| IBIS File LibisMaker.ibs
| Cadence Design Systems, Inc. 2024
|[Doc Num]	 FPGA-MD-02035 Ver 1.5
[IBIS ver]   4.2
[File name]   lfmxo5.ibs
[File Rev]   2.5.1
[Date]   Mon Jun 15 19:07:13 PDT 2026
[Source]   Lattice Semiconductor 28fdsoi Process
[Notes]   Device: LFMXO5-25
   BBG256   Final
   BBG400   Final
   Device: LFMXO5-100T
   BBG400   Final
   Device: LFMXO5-55T
   BBG400   Final
   Device: LFMXO5-15D
   BBG256   Final
   BBG400   Final
   Device: LFMXO5-55TD
   BBG400   Final
   Device: LFMXO5-55TDQ
   BBG400   Final
   CBG256   Final
   Device: LFMXO5-65TDQ
   BBG400   Final
   Device: LFMXO5-65T
   BBG256   Final
   BBG400   Final
   BBG484   Final
   Device: LFMXO5-65
   BBG256   Final
   BBG400   Final
   BBG484   Final
   Device: LFMXO5-35T
   BBG256   Final
   BBG400   Final
   BBG484   Final
   Device: LFMXO5-35
   BBG256   Final
   BBG400   Final
   BBG484   Final
   Device: LFMXO5-20D
   BBG256   Final
   BBG400   Final
   BBG484   Final
   Device: LFMXO5-20TD
   BBG256   Final
   BBG400   Final
   BBG484   Final
   Device: LFMXO5-20DQ
   BBG256   Final
   BBG400   Final
   BBG484   Final
   Device: LFMXO5-20TDQ
   BBG256   Final
   BBG400   Final
   BBG484   Final
   Device: LFMXO5-30D
   BBG256   Final
   BBG400   Final
   BBG484   Final
   Device: LFMXO5-30TD
   BBG256   Final
   BBG400   Final
   BBG484   Final
   Device: LFMXO5-30DQ
   BBG256   Final
   BBG400   Final
   BBG484   Final
   Device: LFMXO5-30TDQ
   BBG256   Final
   BBG400   Final
   BBG484   Final
   Lattice Semiconductor has worked hard to ensure the
   models below are accurate and complete.  However, the
   data below was generated using simulation of the
   input/output model files for the silicon.  Therefore,
   the data below is for reference and initial design
   purposes only.
   Lattice Semiconductor grants permission to use this
   data for use in printed circuit design using this
   Lattice programmable logic device.  Other use of this
   code, including the selling or duplication of any
   portion is strictly prohibited.
|   NAMING CONVENTION
   The IBIS [Model] header is limited by the specification to a
   total of characters.  With such a set of characters available
   for naming models it becomes important to attempt to
   meaningfully encode the IO standards so they fit within the
   twenty character limit.  It would seem that twenty characters
   would provide room enough for describing IO's.  However, the
   PLD IO structure continues to grow more and more complex.  The
   complexity is making the twenty characters insuffiently
   descriptive.  In order to overcome this issue the naming
   convention described below is implemented to resolve the issue.
The twenty character space is managed as follows:
   bbbvvvsdddprttmaoixx
   b = standard
   v = voltage (x.xx V)
   s = slew code
   d = drive (xx.x ma)
   p = pullmode code
   r = impedance
   t = termination code
   m = mipi hard dphy mode
   o = diff resistor code
   i = diff  current code
   x = reserved
   standard
   LVCMOS   lvc
   LVCMOSH   lvh
   LVCMOSR   lvr
   LVCMOSD   lvd
   LVTTL   lvt
   lvttld   ltd
   sstl_I   ss1
   sstl_II   ss2
   sstld_I   s1d
   sstld_II   s2d
   hsul   hs1
   hsuld   h1d
   hstl_I   hs1
   hstld_I   h1d
   lvds   lvs
   lvdse   lve
   SUBLVDS   slv
   sublvdse   sle
   sublvdseh   slh
   slvs   svs
   mipi   mip
   vref1   vr1
   lvstl_I   ll1
   lvstl_II   ll2
   lvstld_I   l1d
   lvstld_II   l2d
   slew
   na   a
   fast   f
   slow   s
   med   m
   drive
   2   020
   4   040
   6   060
   8   080
   10   100
   12   120
   16   160
   50rs   r50
   na   xxx
   pullmode/clamp on
   none   a/e
   failsafe   a/e
   up   b/f
   down   c/g
   keeper   d/h
   i3c   i
   impedance
   off   a
   termination
   off   aa
   40   bb
   50   cc
   60   dd
   75   ee
   150   ff
   48   gg
   80   hh
   120   ii
   mipi hard dphy mode
   off   a
   lp   l
   hs   h
   differential resistor
   off   a
   100   b
   differential current
   NA   a
   2.0   b
   3.5   c
   Reserved   IO type
   in   input only (mipi: rx)
   ou   output (mipi: tx)
   io   I/O
   od   Open drain
   ic   Inverting differential input
   (signal name only)
   it   Non-Inverting differential
   input (signal name only)
   on   Inverting differential output
   (signal name only)
   op   Non-Inverting differential output
   (signal name only)
   bn   Inverting differential I/O
   (signal name only)
   bp   Non-Inverting differential I/O
   (signal name only)
   All the IO models are generated with pull mode set to none.
   Lattice Semiconductor Corporation
   5555 NE Moore Court
   Hillsboro, OR 97214
   U.S.A
   TEL: 1-800-Lattice (USA and Canada)
   408-826-6000 (other locations)
   web: http://www.latticesemi.com/
   email: techsupport@latticesemi.com
[Disclaimer] This IBIS source code is intended as a design reference
   which illustrates how the Lattice Semiconductor device operates.
   It is the user's responsibility to verify their design for
   consistency and functionality through the use of formal
   verification methods.  Lattice Semiconductor provides no warranty
   regarding the use or functionality of this data.
[Copyright]   Copyright 2025 by Lattice Semiconductor Corporation
|   Component LFMXO5
[Component] LFMXO5
[Manufacturer] Lattice Semiconductor Corp.
[Package]
|BBG400_15D
| variable   typ   min   max
R_pkg   0.36549   0.21269   0.57866
L_pkg   3.644e-9   2.134e-9   6.024e-9
C_pkg   1.195e-12   7.084e-13   1.745e-12
|BBG400_15D-AQA
| variable   typ   min   max
|R_pkg   0.36549   0.21269   0.57866
|L_pkg   3.644e-9   2.134e-9   6.024e-9
|C_pkg   1.195e-12   7.084e-13   1.745e-12
|BBG400_15D-HBN
| variable   typ   min   max
|R_pkg   0.36549   0.21269   0.57866
|L_pkg   3.644e-9   2.134e-9   6.024e-9
|C_pkg   1.195e-12   7.084e-13   1.745e-12
|BBG256_15D
| variable   typ   min   max
|R_pkg   0.31029   0.20925   0.48462
|L_pkg   3.215e-9   2.242e-9   4.974e-9
|C_pkg   1.086e-12   7.406e-13   1.53e-12
|BBG400_25
| variable   typ   min   max
|R_pkg   0.36549   0.21269   0.57866
|L_pkg   3.644e-9   2.134e-9   6.024e-9
|C_pkg   1.195e-12   7.084e-13   1.745e-12
|BBG256_25
| variable   typ   min   max
|R_pkg   0.31029   0.20925   0.48462
|L_pkg   3.215e-9   2.242e-9   4.974e-9
|C_pkg   1.086e-12   7.406e-13   1.53e-12
|BBG256_35
| variable   typ   min   max
|R_pkg   0.36575   0.16548   0.7091
|L_pkg   3.369e-9   1.878e-9   5.893e-9
|C_pkg   1.068e-12   6.45e-13   1.798e-12
|BBG256_35T
| variable   typ   min   max
|R_pkg   0.36575   0.16548   0.7091
|L_pkg   3.369e-9   1.878e-9   5.893e-9
|C_pkg   1.068e-12   6.45e-13   1.798e-12
|BBG256_65
| variable   typ   min   max
|R_pkg   0.36575   0.16548   0.7091
|L_pkg   3.369e-9   1.878e-9   5.893e-9
|C_pkg   1.068e-12   6.45e-13   1.798e-12
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[Pin]  signal_name   model_name   R_pin   L_pin   C_pin
1   lvt330f020eaaaaaaaio   lvt330f020eaaaaaaaio
2   lvt330f020faaaaaaaio   lvt330f020faaaaaaaio
3   lvt330f020gaaaaaaaio   lvt330f020gaaaaaaaio
4   lvt330f020haaaaaaaio   lvt330f020haaaaaaaio
5   lvt330f040eaaaaaaaio   lvt330f040eaaaaaaaio
6   lvt330f040faaaaaaaio   lvt330f040faaaaaaaio
7   lvt330f040gaaaaaaaio   lvt330f040gaaaaaaaio
8   lvt330f040haaaaaaaio   lvt330f040haaaaaaaio
9   lvt330f080eaaaaaaaio   lvt330f080eaaaaaaaio
10   lvt330f080faaaaaaaio   lvt330f080faaaaaaaio
11   lvt330f080gaaaaaaaio   lvt330f080gaaaaaaaio
12   lvt330f080haaaaaaaio   lvt330f080haaaaaaaio
13   lvt330f120eaaaaaaaio   lvt330f120eaaaaaaaio
14   lvt330f120faaaaaaaio   lvt330f120faaaaaaaio
15   lvt330f120gaaaaaaaio   lvt330f120gaaaaaaaio
16   lvt330f120haaaaaaaio   lvt330f120haaaaaaaio
17   lvt330f160eaaaaaaaio   lvt330f160eaaaaaaaio
18   lvt330f160faaaaaaaio   lvt330f160faaaaaaaio
19   lvt330f160gaaaaaaaio   lvt330f160gaaaaaaaio
20   lvt330f160haaaaaaaio   lvt330f160haaaaaaaio
21   lvt330fr50eaaaaaaaio   lvt330fr50eaaaaaaaio
22   lvt330fr50faaaaaaaio   lvt330fr50faaaaaaaio
23   lvt330fr50gaaaaaaaio   lvt330fr50gaaaaaaaio
24   lvt330fr50haaaaaaaio   lvt330fr50haaaaaaaio
25   lvt330m020eaaaaaaaio   lvt330m020eaaaaaaaio
26   lvt330m020faaaaaaaio   lvt330m020faaaaaaaio
27   lvt330m020gaaaaaaaio   lvt330m020gaaaaaaaio
28   lvt330m020haaaaaaaio   lvt330m020haaaaaaaio
29   lvt330m040eaaaaaaaio   lvt330m040eaaaaaaaio
30   lvt330m040faaaaaaaio   lvt330m040faaaaaaaio
31   lvt330m040gaaaaaaaio   lvt330m040gaaaaaaaio
32   lvt330m040haaaaaaaio   lvt330m040haaaaaaaio
33   lvt330m080eaaaaaaaio   lvt330m080eaaaaaaaio
34   lvt330m080faaaaaaaio   lvt330m080faaaaaaaio
35   lvt330m080gaaaaaaaio   lvt330m080gaaaaaaaio
36   lvt330m080haaaaaaaio   lvt330m080haaaaaaaio
37   lvt330m120eaaaaaaaio   lvt330m120eaaaaaaaio
38   lvt330m120faaaaaaaio   lvt330m120faaaaaaaio
39   lvt330m120gaaaaaaaio   lvt330m120gaaaaaaaio
40   lvt330m120haaaaaaaio   lvt330m120haaaaaaaio
41   lvt330m160eaaaaaaaio   lvt330m160eaaaaaaaio
42   lvt330m160faaaaaaaio   lvt330m160faaaaaaaio
43   lvt330m160gaaaaaaaio   lvt330m160gaaaaaaaio
44   lvt330m160haaaaaaaio   lvt330m160haaaaaaaio
45   lvt330mr50eaaaaaaaio   lvt330mr50eaaaaaaaio
46   lvt330mr50faaaaaaaio   lvt330mr50faaaaaaaio
47   lvt330mr50gaaaaaaaio   lvt330mr50gaaaaaaaio
48   lvt330mr50haaaaaaaio   lvt330mr50haaaaaaaio
49   lvt330s020eaaaaaaaio   lvt330s020eaaaaaaaio
50   lvt330s020faaaaaaaio   lvt330s020faaaaaaaio
51   lvt330s020gaaaaaaaio   lvt330s020gaaaaaaaio
52   lvt330s020haaaaaaaio   lvt330s020haaaaaaaio
53   lvt330s040eaaaaaaaio   lvt330s040eaaaaaaaio
54   lvt330s040faaaaaaaio   lvt330s040faaaaaaaio
55   lvt330s040gaaaaaaaio   lvt330s040gaaaaaaaio
56   lvt330s040haaaaaaaio   lvt330s040haaaaaaaio
57   lvt330s080eaaaaaaaio   lvt330s080eaaaaaaaio
58   lvt330s080faaaaaaaio   lvt330s080faaaaaaaio
59   lvt330s080gaaaaaaaio   lvt330s080gaaaaaaaio
60   lvt330s080haaaaaaaio   lvt330s080haaaaaaaio
61   lvt330s120eaaaaaaaio   lvt330s120eaaaaaaaio
62   lvt330s120faaaaaaaio   lvt330s120faaaaaaaio
63   lvt330s120gaaaaaaaio   lvt330s120gaaaaaaaio
64   lvt330s120haaaaaaaio   lvt330s120haaaaaaaio
65   lvt330s160eaaaaaaaio   lvt330s160eaaaaaaaio
66   lvt330s160faaaaaaaio   lvt330s160faaaaaaaio
67   lvt330s160gaaaaaaaio   lvt330s160gaaaaaaaio
68   lvt330s160haaaaaaaio   lvt330s160haaaaaaaio
69   lvt330sr50eaaaaaaaio   lvt330sr50eaaaaaaaio
70   lvt330sr50faaaaaaaio   lvt330sr50faaaaaaaio
71   lvt330sr50gaaaaaaaio   lvt330sr50gaaaaaaaio
72   lvt330sr50haaaaaaaio   lvt330sr50haaaaaaaio
73   lvt330f020aaaaaaaaod   lvt330f020aaaaaaaaod
74   lvt330f040aaaaaaaaod   lvt330f040aaaaaaaaod
75   lvt330f080aaaaaaaaod   lvt330f080aaaaaaaaod
76   lvt330f120aaaaaaaaod   lvt330f120aaaaaaaaod
77   lvt330m020aaaaaaaaod   lvt330m020aaaaaaaaod
78   lvt330m040aaaaaaaaod   lvt330m040aaaaaaaaod
79   lvt330m080aaaaaaaaod   lvt330m080aaaaaaaaod
80   lvt330m120aaaaaaaaod   lvt330m120aaaaaaaaod
81   lvt330s020aaaaaaaaod   lvt330s020aaaaaaaaod
82   lvt330s040aaaaaaaaod   lvt330s040aaaaaaaaod
83   lvt330s080aaaaaaaaod   lvt330s080aaaaaaaaod
84   lvt330s120aaaaaaaaod   lvt330s120aaaaaaaaod
85   lvc100axxxaaaaaaaain   lvc100axxxaaaaaaaain
86   lvc100axxxcaaaaaaain   lvc100axxxcaaaaaaain
87   lvc120axxxaaaaaaaain   lvc120axxxaaaaaaaain
88   lvc120axxxbaaaaaaain   lvc120axxxbaaaaaaain
89   lvc120axxxcaaaaaaain   lvc120axxxcaaaaaaain
90   lvc120axxxdaaaaaaain   lvc120axxxdaaaaaaain
91   lvc120axxxiaaaaaaain   lvc120axxxiaaaaaaain
92   lvc150axxxaaaaaaaain   lvc150axxxaaaaaaaain
93   lvc150axxxbaaaaaaain   lvc150axxxbaaaaaaain
94   lvc150axxxcaaaaaaain   lvc150axxxcaaaaaaain
95   lvc150axxxdaaaaaaain   lvc150axxxdaaaaaaain
96   lvc180axxxaaaaaaaain   lvc180axxxaaaaaaaain
97   lvc180axxxcaaaaaaain   lvc180axxxcaaaaaaain
98   lvc180axxxeaaaaaaain   lvc180axxxeaaaaaaain
99   lvc180axxxfaaaaaaain   lvc180axxxfaaaaaaain
100   lvc180axxxgaaaaaaain   lvc180axxxgaaaaaaain
101   lvc180axxxhaaaaaaain   lvc180axxxhaaaaaaain
102   lvc180axxxiaaaaaaain   lvc180axxxiaaaaaaain
103   lvc250axxxaaaaaaaain   lvc250axxxaaaaaaaain
104   lvc250axxxcaaaaaaain   lvc250axxxcaaaaaaain
105   lvc250axxxeaaaaaaain   lvc250axxxeaaaaaaain
106   lvc250axxxfaaaaaaain   lvc250axxxfaaaaaaain
107   lvc250axxxgaaaaaaain   lvc250axxxgaaaaaaain
108   lvc250axxxhaaaaaaain   lvc250axxxhaaaaaaain
109   lvc250axxxiaaaaaaain   lvc250axxxiaaaaaaain
110   lvc330axxxeaaaaaaain   lvc330axxxeaaaaaaain
111   lvc330axxxfaaaaaaain   lvc330axxxfaaaaaaain
112   lvc330axxxgaaaaaaain   lvc330axxxgaaaaaaain
113   lvc330axxxhaaaaaaain   lvc330axxxhaaaaaaain
114   lvc330axxxiaaaaaaain   lvc330axxxiaaaaaaain
115   lvt330axxxeaaaaaaain   lvt330axxxeaaaaaaain
116   lvt330axxxfaaaaaaain   lvt330axxxfaaaaaaain
117   lvt330axxxgaaaaaaain   lvt330axxxgaaaaaaain
118   lvt330axxxhaaaaaaain   lvt330axxxhaaaaaaain
119   lvc120f020aaaaaaaaio   lvc120f020aaaaaaaaio
120   lvc120f020baaaaaaaio   lvc120f020baaaaaaaio
121   lvc120f020caaaaaaaio   lvc120f020caaaaaaaio
122   lvc120f020daaaaaaaio   lvc120f020daaaaaaaio
123   lvc120f020iaaaaaaaio   lvc120f020iaaaaaaaio
124   lvc120f040aaaaaaaaio   lvc120f040aaaaaaaaio
125   lvc120f040baaaaaaaio   lvc120f040baaaaaaaio
126   lvc120f040caaaaaaaio   lvc120f040caaaaaaaio
127   lvc120f040daaaaaaaio   lvc120f040daaaaaaaio
128   lvc120f040iaaaaaaaio   lvc120f040iaaaaaaaio
129   lvc120m020aaaaaaaaio   lvc120m020aaaaaaaaio
130   lvc120m020baaaaaaaio   lvc120m020baaaaaaaio
131   lvc120m020caaaaaaaio   lvc120m020caaaaaaaio
132   lvc120m020daaaaaaaio   lvc120m020daaaaaaaio
133   lvc120m020iaaaaaaaio   lvc120m020iaaaaaaaio
134   lvc120m040aaaaaaaaio   lvc120m040aaaaaaaaio
135   lvc120m040baaaaaaaio   lvc120m040baaaaaaaio
136   lvc120m040caaaaaaaio   lvc120m040caaaaaaaio
137   lvc120m040daaaaaaaio   lvc120m040daaaaaaaio
138   lvc120m040iaaaaaaaio   lvc120m040iaaaaaaaio
139   lvc120s020aaaaaaaaio   lvc120s020aaaaaaaaio
140   lvc120s020baaaaaaaio   lvc120s020baaaaaaaio
141   lvc120s020caaaaaaaio   lvc120s020caaaaaaaio
142   lvc120s020daaaaaaaio   lvc120s020daaaaaaaio
143   lvc120s020iaaaaaaaio   lvc120s020iaaaaaaaio
144   lvc120s040aaaaaaaaio   lvc120s040aaaaaaaaio
145   lvc120s040baaaaaaaio   lvc120s040baaaaaaaio
146   lvc120s040caaaaaaaio   lvc120s040caaaaaaaio
147   lvc120s040daaaaaaaio   lvc120s040daaaaaaaio
148   lvc120s040iaaaaaaaio   lvc120s040iaaaaaaaio
149   lvc150f020aaaaaaaaio   lvc150f020aaaaaaaaio
150   lvc150f020baaaaaaaio   lvc150f020baaaaaaaio
151   lvc150f020caaaaaaaio   lvc150f020caaaaaaaio
152   lvc150f020daaaaaaaio   lvc150f020daaaaaaaio
153   lvc150f040aaaaaaaaio   lvc150f040aaaaaaaaio
154   lvc150f040baaaaaaaio   lvc150f040baaaaaaaio
155   lvc150f040caaaaaaaio   lvc150f040caaaaaaaio
156   lvc150f040daaaaaaaio   lvc150f040daaaaaaaio
157   lvc150m020aaaaaaaaio   lvc150m020aaaaaaaaio
158   lvc150m020baaaaaaaio   lvc150m020baaaaaaaio
159   lvc150m020caaaaaaaio   lvc150m020caaaaaaaio
160   lvc150m020daaaaaaaio   lvc150m020daaaaaaaio
161   lvc150m040aaaaaaaaio   lvc150m040aaaaaaaaio
162   lvc150m040baaaaaaaio   lvc150m040baaaaaaaio
163   lvc150m040caaaaaaaio   lvc150m040caaaaaaaio
164   lvc150m040daaaaaaaio   lvc150m040daaaaaaaio
165   lvc150s020aaaaaaaaio   lvc150s020aaaaaaaaio
166   lvc150s020baaaaaaaio   lvc150s020baaaaaaaio
167   lvc150s020caaaaaaaio   lvc150s020caaaaaaaio
168   lvc150s020daaaaaaaio   lvc150s020daaaaaaaio
169   lvc150s040aaaaaaaaio   lvc150s040aaaaaaaaio
170   lvc150s040baaaaaaaio   lvc150s040baaaaaaaio
171   lvc150s040caaaaaaaio   lvc150s040caaaaaaaio
172   lvc150s040daaaaaaaio   lvc150s040daaaaaaaio
173   lvc180f020aaaaaaaaio   lvc180f020aaaaaaaaio
174   lvc180f020baaaaaaaio   lvc180f020baaaaaaaio
175   lvc180f020caaaaaaaio   lvc180f020caaaaaaaio
176   lvc180f020daaaaaaaio   lvc180f020daaaaaaaio
177   lvc180f020iaaaaaaaio   lvc180f020iaaaaaaaio
178   lvc180f040aaaaaaaaio   lvc180f040aaaaaaaaio
179   lvc180f040baaaaaaaio   lvc180f040baaaaaaaio
180   lvc180f040caaaaaaaio   lvc180f040caaaaaaaio
181   lvc180f040daaaaaaaio   lvc180f040daaaaaaaio
182   lvc180f040iaaaaaaaio   lvc180f040iaaaaaaaio
183   lvc180f080aaaaaaaaio   lvc180f080aaaaaaaaio
184   lvc180f080baaaaaaaio   lvc180f080baaaaaaaio
185   lvc180f080caaaaaaaio   lvc180f080caaaaaaaio
186   lvc180f080daaaaaaaio   lvc180f080daaaaaaaio
187   lvc180f080iaaaaaaaio   lvc180f080iaaaaaaaio
188   lvc180fr50aaaaaaaaio   lvc180fr50aaaaaaaaio
189   lvc180fr50baaaaaaaio   lvc180fr50baaaaaaaio
190   lvc180fr50caaaaaaaio   lvc180fr50caaaaaaaio
191   lvc180fr50daaaaaaaio   lvc180fr50daaaaaaaio
192   lvc180fr50iaaaaaaaio   lvc180fr50iaaaaaaaio
193   lvc180m020aaaaaaaaio   lvc180m020aaaaaaaaio
194   lvc180m020baaaaaaaio   lvc180m020baaaaaaaio
195   lvc180m020caaaaaaaio   lvc180m020caaaaaaaio
196   lvc180m020daaaaaaaio   lvc180m020daaaaaaaio
197   lvc180m020iaaaaaaaio   lvc180m020iaaaaaaaio
198   lvc180m040aaaaaaaaio   lvc180m040aaaaaaaaio
199   lvc180m040baaaaaaaio   lvc180m040baaaaaaaio
200   lvc180m040caaaaaaaio   lvc180m040caaaaaaaio
201   lvc180m040daaaaaaaio   lvc180m040daaaaaaaio
202   lvc180m040iaaaaaaaio   lvc180m040iaaaaaaaio
203   lvc180m080aaaaaaaaio   lvc180m080aaaaaaaaio
204   lvc180m080baaaaaaaio   lvc180m080baaaaaaaio
205   lvc180m080caaaaaaaio   lvc180m080caaaaaaaio
206   lvc180m080daaaaaaaio   lvc180m080daaaaaaaio
207   lvc180m080iaaaaaaaio   lvc180m080iaaaaaaaio
208   lvc180mr50aaaaaaaaio   lvc180mr50aaaaaaaaio
209   lvc180mr50baaaaaaaio   lvc180mr50baaaaaaaio
210   lvc180mr50caaaaaaaio   lvc180mr50caaaaaaaio
211   lvc180mr50daaaaaaaio   lvc180mr50daaaaaaaio
212   lvc180mr50iaaaaaaaio   lvc180mr50iaaaaaaaio
213   lvc180s020aaaaaaaaio   lvc180s020aaaaaaaaio
214   lvc180s020baaaaaaaio   lvc180s020baaaaaaaio
215   lvc180s020caaaaaaaio   lvc180s020caaaaaaaio
216   lvc180s020daaaaaaaio   lvc180s020daaaaaaaio
217   lvc180s020iaaaaaaaio   lvc180s020iaaaaaaaio
218   lvc180s040aaaaaaaaio   lvc180s040aaaaaaaaio
219   lvc180s040baaaaaaaio   lvc180s040baaaaaaaio
220   lvc180s040caaaaaaaio   lvc180s040caaaaaaaio
221   lvc180s040daaaaaaaio   lvc180s040daaaaaaaio
222   lvc180s040iaaaaaaaio   lvc180s040iaaaaaaaio
223   lvc180s080aaaaaaaaio   lvc180s080aaaaaaaaio
224   lvc180s080baaaaaaaio   lvc180s080baaaaaaaio
225   lvc180s080caaaaaaaio   lvc180s080caaaaaaaio
226   lvc180s080daaaaaaaio   lvc180s080daaaaaaaio
227   lvc180s080iaaaaaaaio   lvc180s080iaaaaaaaio
228   lvc180sr50aaaaaaaaio   lvc180sr50aaaaaaaaio
229   lvc180sr50baaaaaaaio   lvc180sr50baaaaaaaio
230   lvc180sr50caaaaaaaio   lvc180sr50caaaaaaaio
231   lvc180sr50daaaaaaaio   lvc180sr50daaaaaaaio
232   lvc180sr50iaaaaaaaio   lvc180sr50iaaaaaaaio
233   lvc250f020eaaaaaaaio   lvc250f020eaaaaaaaio
234   lvc250f020faaaaaaaio   lvc250f020faaaaaaaio
235   lvc250f020gaaaaaaaio   lvc250f020gaaaaaaaio
236   lvc250f020haaaaaaaio   lvc250f020haaaaaaaio
237   lvc250f020iaaaaaaaio   lvc250f020iaaaaaaaio
238   lvc250f040eaaaaaaaio   lvc250f040eaaaaaaaio
239   lvc250f040faaaaaaaio   lvc250f040faaaaaaaio
240   lvc250f040gaaaaaaaio   lvc250f040gaaaaaaaio
241   lvc250f040haaaaaaaio   lvc250f040haaaaaaaio
242   lvc250f040iaaaaaaaio   lvc250f040iaaaaaaaio
243   lvc250f080eaaaaaaaio   lvc250f080eaaaaaaaio
244   lvc250f080faaaaaaaio   lvc250f080faaaaaaaio
245   lvc250f080gaaaaaaaio   lvc250f080gaaaaaaaio
246   lvc250f080haaaaaaaio   lvc250f080haaaaaaaio
247   lvc250f080iaaaaaaaio   lvc250f080iaaaaaaaio
248   lvc250f100eaaaaaaaio   lvc250f100eaaaaaaaio
249   lvc250f100faaaaaaaio   lvc250f100faaaaaaaio
250   lvc250f100gaaaaaaaio   lvc250f100gaaaaaaaio
251   lvc250f100haaaaaaaio   lvc250f100haaaaaaaio
252   lvc250f100iaaaaaaaio   lvc250f100iaaaaaaaio
253   lvc250fr50eaaaaaaaio   lvc250fr50eaaaaaaaio
254   lvc250fr50faaaaaaaio   lvc250fr50faaaaaaaio
255   lvc250fr50gaaaaaaaio   lvc250fr50gaaaaaaaio
256   lvc250fr50haaaaaaaio   lvc250fr50haaaaaaaio
257   lvc250fr50iaaaaaaaio   lvc250fr50iaaaaaaaio
258   lvc250m020eaaaaaaaio   lvc250m020eaaaaaaaio
259   lvc250m020faaaaaaaio   lvc250m020faaaaaaaio
260   lvc250m020gaaaaaaaio   lvc250m020gaaaaaaaio
261   lvc250m020haaaaaaaio   lvc250m020haaaaaaaio
262   lvc250m020iaaaaaaaio   lvc250m020iaaaaaaaio
263   lvc250m040eaaaaaaaio   lvc250m040eaaaaaaaio
264   lvc250m040faaaaaaaio   lvc250m040faaaaaaaio
265   lvc250m040gaaaaaaaio   lvc250m040gaaaaaaaio
266   lvc250m040haaaaaaaio   lvc250m040haaaaaaaio
267   lvc250m040iaaaaaaaio   lvc250m040iaaaaaaaio
268   lvc250m080eaaaaaaaio   lvc250m080eaaaaaaaio
269   lvc250m080faaaaaaaio   lvc250m080faaaaaaaio
270   lvc250m080gaaaaaaaio   lvc250m080gaaaaaaaio
271   lvc250m080haaaaaaaio   lvc250m080haaaaaaaio
272   lvc250m080iaaaaaaaio   lvc250m080iaaaaaaaio
273   lvc250m100eaaaaaaaio   lvc250m100eaaaaaaaio
274   lvc250m100faaaaaaaio   lvc250m100faaaaaaaio
275   lvc250m100gaaaaaaaio   lvc250m100gaaaaaaaio
276   lvc250m100haaaaaaaio   lvc250m100haaaaaaaio
277   lvc250m100iaaaaaaaio   lvc250m100iaaaaaaaio
278   lvc250mr50eaaaaaaaio   lvc250mr50eaaaaaaaio
279   lvc250mr50faaaaaaaio   lvc250mr50faaaaaaaio
280   lvc250mr50gaaaaaaaio   lvc250mr50gaaaaaaaio
281   lvc250mr50haaaaaaaio   lvc250mr50haaaaaaaio
282   lvc250mr50iaaaaaaaio   lvc250mr50iaaaaaaaio
283   lvc250s020eaaaaaaaio   lvc250s020eaaaaaaaio
284   lvc250s020faaaaaaaio   lvc250s020faaaaaaaio
285   lvc250s020gaaaaaaaio   lvc250s020gaaaaaaaio
286   lvc250s020haaaaaaaio   lvc250s020haaaaaaaio
287   lvc250s020iaaaaaaaio   lvc250s020iaaaaaaaio
288   lvc250s040eaaaaaaaio   lvc250s040eaaaaaaaio
289   lvc250s040faaaaaaaio   lvc250s040faaaaaaaio
290   lvc250s040gaaaaaaaio   lvc250s040gaaaaaaaio
291   lvc250s040haaaaaaaio   lvc250s040haaaaaaaio
292   lvc250s040iaaaaaaaio   lvc250s040iaaaaaaaio
293   lvc250s080eaaaaaaaio   lvc250s080eaaaaaaaio
294   lvc250s080faaaaaaaio   lvc250s080faaaaaaaio
295   lvc250s080gaaaaaaaio   lvc250s080gaaaaaaaio
296   lvc250s080haaaaaaaio   lvc250s080haaaaaaaio
297   lvc250s080iaaaaaaaio   lvc250s080iaaaaaaaio
298   lvc250s100eaaaaaaaio   lvc250s100eaaaaaaaio
299   lvc250s100faaaaaaaio   lvc250s100faaaaaaaio
300   lvc250s100gaaaaaaaio   lvc250s100gaaaaaaaio
301   lvc250s100haaaaaaaio   lvc250s100haaaaaaaio
302   lvc250s100iaaaaaaaio   lvc250s100iaaaaaaaio
303   lvc250sr50eaaaaaaaio   lvc250sr50eaaaaaaaio
304   lvc250sr50faaaaaaaio   lvc250sr50faaaaaaaio
305   lvc250sr50gaaaaaaaio   lvc250sr50gaaaaaaaio
306   lvc250sr50haaaaaaaio   lvc250sr50haaaaaaaio
307   lvc250sr50iaaaaaaaio   lvc250sr50iaaaaaaaio
308   lvc330f020eaaaaaaaio   lvc330f020eaaaaaaaio
309   lvc330f020faaaaaaaio   lvc330f020faaaaaaaio
310   lvc330f020gaaaaaaaio   lvc330f020gaaaaaaaio
311   lvc330f020haaaaaaaio   lvc330f020haaaaaaaio
312   lvc330f020iaaaaaaaio   lvc330f020iaaaaaaaio
313   lvc330f040eaaaaaaaio   lvc330f040eaaaaaaaio
314   lvc330f040faaaaaaaio   lvc330f040faaaaaaaio
315   lvc330f040gaaaaaaaio   lvc330f040gaaaaaaaio
316   lvc330f040haaaaaaaio   lvc330f040haaaaaaaio
317   lvc330f040iaaaaaaaio   lvc330f040iaaaaaaaio
318   lvc330f080eaaaaaaaio   lvc330f080eaaaaaaaio
319   lvc330f080faaaaaaaio   lvc330f080faaaaaaaio
320   lvc330f080gaaaaaaaio   lvc330f080gaaaaaaaio
321   lvc330f080haaaaaaaio   lvc330f080haaaaaaaio
322   lvc330f080iaaaaaaaio   lvc330f080iaaaaaaaio
323   lvc330f120eaaaaaaaio   lvc330f120eaaaaaaaio
324   lvc330f120faaaaaaaio   lvc330f120faaaaaaaio
325   lvc330f120gaaaaaaaio   lvc330f120gaaaaaaaio
326   lvc330f120haaaaaaaio   lvc330f120haaaaaaaio
327   lvc330f120iaaaaaaaio   lvc330f120iaaaaaaaio
328   lvc330f160eaaaaaaaio   lvc330f160eaaaaaaaio
329   lvc330f160faaaaaaaio   lvc330f160faaaaaaaio
330   lvc330f160gaaaaaaaio   lvc330f160gaaaaaaaio
331   lvc330f160haaaaaaaio   lvc330f160haaaaaaaio
332   lvc330f160iaaaaaaaio   lvc330f160iaaaaaaaio
333   lvc330fr50eaaaaaaaio   lvc330fr50eaaaaaaaio
334   lvc330fr50faaaaaaaio   lvc330fr50faaaaaaaio
335   lvc330fr50gaaaaaaaio   lvc330fr50gaaaaaaaio
336   lvc330fr50haaaaaaaio   lvc330fr50haaaaaaaio
337   lvc330fr50iaaaaaaaio   lvc330fr50iaaaaaaaio
338   lvc330m020eaaaaaaaio   lvc330m020eaaaaaaaio
339   lvc330m020faaaaaaaio   lvc330m020faaaaaaaio
340   lvc330m020gaaaaaaaio   lvc330m020gaaaaaaaio
341   lvc330m020haaaaaaaio   lvc330m020haaaaaaaio
342   lvc330m020iaaaaaaaio   lvc330m020iaaaaaaaio
343   lvc330m040eaaaaaaaio   lvc330m040eaaaaaaaio
344   lvc330m040faaaaaaaio   lvc330m040faaaaaaaio
345   lvc330m040gaaaaaaaio   lvc330m040gaaaaaaaio
346   lvc330m040haaaaaaaio   lvc330m040haaaaaaaio
347   lvc330m040iaaaaaaaio   lvc330m040iaaaaaaaio
348   lvc330m080eaaaaaaaio   lvc330m080eaaaaaaaio
349   lvc330m080faaaaaaaio   lvc330m080faaaaaaaio
350   lvc330m080gaaaaaaaio   lvc330m080gaaaaaaaio
351   lvc330m080haaaaaaaio   lvc330m080haaaaaaaio
352   lvc330m080iaaaaaaaio   lvc330m080iaaaaaaaio
353   lvc330m120eaaaaaaaio   lvc330m120eaaaaaaaio
354   lvc330m120faaaaaaaio   lvc330m120faaaaaaaio
355   lvc330m120gaaaaaaaio   lvc330m120gaaaaaaaio
356   lvc330m120haaaaaaaio   lvc330m120haaaaaaaio
357   lvc330m120iaaaaaaaio   lvc330m120iaaaaaaaio
358   lvc330m160eaaaaaaaio   lvc330m160eaaaaaaaio
359   lvc330m160faaaaaaaio   lvc330m160faaaaaaaio
360   lvc330m160gaaaaaaaio   lvc330m160gaaaaaaaio
361   lvc330m160haaaaaaaio   lvc330m160haaaaaaaio
362   lvc330m160iaaaaaaaio   lvc330m160iaaaaaaaio
363   lvc330mr50eaaaaaaaio   lvc330mr50eaaaaaaaio
364   lvc330mr50faaaaaaaio   lvc330mr50faaaaaaaio
365   lvc330mr50gaaaaaaaio   lvc330mr50gaaaaaaaio
366   lvc330mr50haaaaaaaio   lvc330mr50haaaaaaaio
367   lvc330mr50iaaaaaaaio   lvc330mr50iaaaaaaaio
368   lvc330s020eaaaaaaaio   lvc330s020eaaaaaaaio
369   lvc330s020faaaaaaaio   lvc330s020faaaaaaaio
370   lvc330s020gaaaaaaaio   lvc330s020gaaaaaaaio
371   lvc330s020haaaaaaaio   lvc330s020haaaaaaaio
372   lvc330s020iaaaaaaaio   lvc330s020iaaaaaaaio
373   lvc330s040eaaaaaaaio   lvc330s040eaaaaaaaio
374   lvc330s040faaaaaaaio   lvc330s040faaaaaaaio
375   lvc330s040gaaaaaaaio   lvc330s040gaaaaaaaio
376   lvc330s040haaaaaaaio   lvc330s040haaaaaaaio
377   lvc330s040iaaaaaaaio   lvc330s040iaaaaaaaio
378   lvc330s080eaaaaaaaio   lvc330s080eaaaaaaaio
379   lvc330s080faaaaaaaio   lvc330s080faaaaaaaio
380   lvc330s080gaaaaaaaio   lvc330s080gaaaaaaaio
381   lvc330s080haaaaaaaio   lvc330s080haaaaaaaio
382   lvc330s080iaaaaaaaio   lvc330s080iaaaaaaaio
383   lvc330s120eaaaaaaaio   lvc330s120eaaaaaaaio
384   lvc330s120faaaaaaaio   lvc330s120faaaaaaaio
385   lvc330s120gaaaaaaaio   lvc330s120gaaaaaaaio
386   lvc330s120haaaaaaaio   lvc330s120haaaaaaaio
387   lvc330s120iaaaaaaaio   lvc330s120iaaaaaaaio
388   lvc330s160eaaaaaaaio   lvc330s160eaaaaaaaio
389   lvc330s160faaaaaaaio   lvc330s160faaaaaaaio
390   lvc330s160gaaaaaaaio   lvc330s160gaaaaaaaio
391   lvc330s160haaaaaaaio   lvc330s160haaaaaaaio
392   lvc330s160iaaaaaaaio   lvc330s160iaaaaaaaio
393   lvc330sr50eaaaaaaaio   lvc330sr50eaaaaaaaio
394   lvc330sr50faaaaaaaio   lvc330sr50faaaaaaaio
395   lvc330sr50gaaaaaaaio   lvc330sr50gaaaaaaaio
396   lvc330sr50haaaaaaaio   lvc330sr50haaaaaaaio
397   lvc330sr50iaaaaaaaio   lvc330sr50iaaaaaaaio
398   lvc120f020aaaaaaaaou   lvc120f020aaaaaaaaou
399   lvc120f040aaaaaaaaou   lvc120f040aaaaaaaaou
400   lvc120m020aaaaaaaaou   lvc120m020aaaaaaaaou
401   lvc120m040aaaaaaaaou   lvc120m040aaaaaaaaou
402   lvc120s020aaaaaaaaou   lvc120s020aaaaaaaaou
403   lvc120s040aaaaaaaaou   lvc120s040aaaaaaaaou
404   lvc150f020aaaaaaaaou   lvc150f020aaaaaaaaou
405   lvc150f040aaaaaaaaou   lvc150f040aaaaaaaaou
406   lvc150m020aaaaaaaaou   lvc150m020aaaaaaaaou
407   lvc150m040aaaaaaaaou   lvc150m040aaaaaaaaou
408   lvc150s020aaaaaaaaou   lvc150s020aaaaaaaaou
409   lvc150s040aaaaaaaaou   lvc150s040aaaaaaaaou
410   lvc180f020aaaaaaaaou   lvc180f020aaaaaaaaou
411   lvc180f040aaaaaaaaou   lvc180f040aaaaaaaaou
412   lvc180f080aaaaaaaaou   lvc180f080aaaaaaaaou
413   lvc180fr50aaaaaaaaou   lvc180fr50aaaaaaaaou
414   lvc180m020aaaaaaaaou   lvc180m020aaaaaaaaou
415   lvc180m040aaaaaaaaou   lvc180m040aaaaaaaaou
416   lvc180m080aaaaaaaaou   lvc180m080aaaaaaaaou
417   lvc180mr50aaaaaaaaou   lvc180mr50aaaaaaaaou
418   lvc180s020aaaaaaaaou   lvc180s020aaaaaaaaou
419   lvc180s040aaaaaaaaou   lvc180s040aaaaaaaaou
420   lvc180s080aaaaaaaaou   lvc180s080aaaaaaaaou
421   lvc180sr50aaaaaaaaou   lvc180sr50aaaaaaaaou
422   lvc250f020aaaaaaaaou   lvc250f020aaaaaaaaou
423   lvc250f040aaaaaaaaou   lvc250f040aaaaaaaaou
424   lvc250f080aaaaaaaaou   lvc250f080aaaaaaaaou
425   lvc250f100aaaaaaaaou   lvc250f100aaaaaaaaou
426   lvc250fr50aaaaaaaaou   lvc250fr50aaaaaaaaou
427   lvc250m020aaaaaaaaou   lvc250m020aaaaaaaaou
428   lvc250m040aaaaaaaaou   lvc250m040aaaaaaaaou
429   lvc250m080aaaaaaaaou   lvc250m080aaaaaaaaou
430   lvc250m100aaaaaaaaou   lvc250m100aaaaaaaaou
431   lvc250mr50aaaaaaaaou   lvc250mr50aaaaaaaaou
432   lvc250s020aaaaaaaaou   lvc250s020aaaaaaaaou
433   lvc250s040aaaaaaaaou   lvc250s040aaaaaaaaou
434   lvc250s080aaaaaaaaou   lvc250s080aaaaaaaaou
435   lvc250s100aaaaaaaaou   lvc250s100aaaaaaaaou
436   lvc250sr50aaaaaaaaou   lvc250sr50aaaaaaaaou
437   lvc330f020aaaaaaaaou   lvc330f020aaaaaaaaou
438   lvc330f040aaaaaaaaou   lvc330f040aaaaaaaaou
439   lvc330f080aaaaaaaaou   lvc330f080aaaaaaaaou
440   lvc330f120aaaaaaaaou   lvc330f120aaaaaaaaou
441   lvc330f160aaaaaaaaou   lvc330f160aaaaaaaaou
442   lvc330fr50aaaaaaaaou   lvc330fr50aaaaaaaaou
443   lvc330m020aaaaaaaaou   lvc330m020aaaaaaaaou
444   lvc330m040aaaaaaaaou   lvc330m040aaaaaaaaou
445   lvc330m080aaaaaaaaou   lvc330m080aaaaaaaaou
446   lvc330m120aaaaaaaaou   lvc330m120aaaaaaaaou
447   lvc330m160aaaaaaaaou   lvc330m160aaaaaaaaou
448   lvc330mr50aaaaaaaaou   lvc330mr50aaaaaaaaou
449   lvc330s020aaaaaaaaou   lvc330s020aaaaaaaaou
450   lvc330s040aaaaaaaaou   lvc330s040aaaaaaaaou
451   lvc330s080aaaaaaaaou   lvc330s080aaaaaaaaou
452   lvc330s120aaaaaaaaou   lvc330s120aaaaaaaaou
453   lvc330s160aaaaaaaaou   lvc330s160aaaaaaaaou
454   lvc330sr50aaaaaaaaou   lvc330sr50aaaaaaaaou
455   lvc120f020aaaaaaaaod   lvc120f020aaaaaaaaod
456   lvc120f040aaaaaaaaod   lvc120f040aaaaaaaaod
457   lvc120m020aaaaaaaaod   lvc120m020aaaaaaaaod
458   lvc120m040aaaaaaaaod   lvc120m040aaaaaaaaod
459   lvc120s020aaaaaaaaod   lvc120s020aaaaaaaaod
460   lvc120s040aaaaaaaaod   lvc120s040aaaaaaaaod
461   lvc150f020aaaaaaaaod   lvc150f020aaaaaaaaod
462   lvc150f040aaaaaaaaod   lvc150f040aaaaaaaaod
463   lvc150m020aaaaaaaaod   lvc150m020aaaaaaaaod
464   lvc150m040aaaaaaaaod   lvc150m040aaaaaaaaod
465   lvc150s020aaaaaaaaod   lvc150s020aaaaaaaaod
466   lvc150s040aaaaaaaaod   lvc150s040aaaaaaaaod
467   lvc180f020aaaaaaaaod   lvc180f020aaaaaaaaod
468   lvc180f040aaaaaaaaod   lvc180f040aaaaaaaaod
469   lvc180f080aaaaaaaaod   lvc180f080aaaaaaaaod
470   lvc180m020aaaaaaaaod   lvc180m020aaaaaaaaod
471   lvc180m040aaaaaaaaod   lvc180m040aaaaaaaaod
472   lvc180m080aaaaaaaaod   lvc180m080aaaaaaaaod
473   lvc180s020aaaaaaaaod   lvc180s020aaaaaaaaod
474   lvc180s040aaaaaaaaod   lvc180s040aaaaaaaaod
475   lvc180s080aaaaaaaaod   lvc180s080aaaaaaaaod
476   lvc250f020aaaaaaaaod   lvc250f020aaaaaaaaod
477   lvc250f040aaaaaaaaod   lvc250f040aaaaaaaaod
478   lvc250f080aaaaaaaaod   lvc250f080aaaaaaaaod
479   lvc250f100aaaaaaaaod   lvc250f100aaaaaaaaod
480   lvc250m020aaaaaaaaod   lvc250m020aaaaaaaaod
481   lvc250m040aaaaaaaaod   lvc250m040aaaaaaaaod
482   lvc250m080aaaaaaaaod   lvc250m080aaaaaaaaod
483   lvc250m100aaaaaaaaod   lvc250m100aaaaaaaaod
484   lvc250s020aaaaaaaaod   lvc250s020aaaaaaaaod
485   lvc250s040aaaaaaaaod   lvc250s040aaaaaaaaod
486   lvc250s080aaaaaaaaod   lvc250s080aaaaaaaaod
487   lvc250s100aaaaaaaaod   lvc250s100aaaaaaaaod
488   lvc330f020aaaaaaaaod   lvc330f020aaaaaaaaod
489   lvc330f040aaaaaaaaod   lvc330f040aaaaaaaaod
490   lvc330f080aaaaaaaaod   lvc330f080aaaaaaaaod
491   lvc330f120aaaaaaaaod   lvc330f120aaaaaaaaod
492   lvc330m020aaaaaaaaod   lvc330m020aaaaaaaaod
493   lvc330m040aaaaaaaaod   lvc330m040aaaaaaaaod
494   lvc330m080aaaaaaaaod   lvc330m080aaaaaaaaod
495   lvc330m120aaaaaaaaod   lvc330m120aaaaaaaaod
496   lvc330s020aaaaaaaaod   lvc330s020aaaaaaaaod
497   lvc330s040aaaaaaaaod   lvc330s040aaaaaaaaod
498   lvc330s080aaaaaaaaod   lvc330s080aaaaaaaaod
499   lvc330s120aaaaaaaaod   lvc330s120aaaaaaaaod
500   sle180f080eaaaaaaaop   sle180f080eaaaaaaaou
501   sle180f080eaaaaaaaon   sle180f080eaaaaaaaou
502   sle180m080eaaaaaaaop   sle180m080eaaaaaaaou
503   sle180m080eaaaaaaaon   sle180m080eaaaaaaaou
504   lvd250f020aaaaaaaaop   lvd250f020aaaaaaaaou
505   lvd250f020aaaaaaaaon   lvd250f020aaaaaaaaou
506   lvd250f040aaaaaaaaop   lvd250f040aaaaaaaaou
507   lvd250f040aaaaaaaaon   lvd250f040aaaaaaaaou
508   lvd250f080aaaaaaaaop   lvd250f080aaaaaaaaou
509   lvd250f080aaaaaaaaon   lvd250f080aaaaaaaaou
510   lvd250f100aaaaaaaaop   lvd250f100aaaaaaaaou
511   lvd250f100aaaaaaaaon   lvd250f100aaaaaaaaou
512   lvd250fr50aaaaaaaaop   lvd250fr50aaaaaaaaou
513   lvd250fr50aaaaaaaaon   lvd250fr50aaaaaaaaou
514   lvd250m020aaaaaaaaop   lvd250m020aaaaaaaaou
515   lvd250m020aaaaaaaaon   lvd250m020aaaaaaaaou
516   lvd250m040aaaaaaaaop   lvd250m040aaaaaaaaou
517   lvd250m040aaaaaaaaon   lvd250m040aaaaaaaaou
518   lvd250m080aaaaaaaaop   lvd250m080aaaaaaaaou
519   lvd250m080aaaaaaaaon   lvd250m080aaaaaaaaou
520   lvd250m100aaaaaaaaop   lvd250m100aaaaaaaaou
521   lvd250m100aaaaaaaaon   lvd250m100aaaaaaaaou
522   lvd250mr50aaaaaaaaop   lvd250mr50aaaaaaaaou
523   lvd250mr50aaaaaaaaon   lvd250mr50aaaaaaaaou
524   lvd250s020aaaaaaaaop   lvd250s020aaaaaaaaou
525   lvd250s020aaaaaaaaon   lvd250s020aaaaaaaaou
526   lvd250s040aaaaaaaaop   lvd250s040aaaaaaaaou
527   lvd250s040aaaaaaaaon   lvd250s040aaaaaaaaou
528   lvd250s080aaaaaaaaop   lvd250s080aaaaaaaaou
529   lvd250s080aaaaaaaaon   lvd250s080aaaaaaaaou
530   lvd250s100aaaaaaaaop   lvd250s100aaaaaaaaou
531   lvd250s100aaaaaaaaon   lvd250s100aaaaaaaaou
532   lvd250sr50aaaaaaaaop   lvd250sr50aaaaaaaaou
533   lvd250sr50aaaaaaaaon   lvd250sr50aaaaaaaaou
534   lve250f080eaaaaaaaop   lve250f080eaaaaaaaou
535   lve250f080eaaaaaaaon   lve250f080eaaaaaaaou
536   lve250m080eaaaaaaaop   lve250m080eaaaaaaaou
537   lve250m080eaaaaaaaon   lve250m080eaaaaaaaou
538   ltd330f020aaaaaaaaop   ltd330f020aaaaaaaaou
539   ltd330f020aaaaaaaaon   ltd330f020aaaaaaaaou
540   ltd330f040aaaaaaaaop   ltd330f040aaaaaaaaou
541   ltd330f040aaaaaaaaon   ltd330f040aaaaaaaaou
542   ltd330f080aaaaaaaaop   ltd330f080aaaaaaaaou
543   ltd330f080aaaaaaaaon   ltd330f080aaaaaaaaou
544   ltd330f120aaaaaaaaop   ltd330f120aaaaaaaaou
545   ltd330f120aaaaaaaaon   ltd330f120aaaaaaaaou
546   ltd330fr50aaaaaaaaop   ltd330fr50aaaaaaaaou
547   ltd330fr50aaaaaaaaon   ltd330fr50aaaaaaaaou
548   ltd330m020aaaaaaaaop   ltd330m020aaaaaaaaou
549   ltd330m020aaaaaaaaon   ltd330m020aaaaaaaaou
550   ltd330m040aaaaaaaaop   ltd330m040aaaaaaaaou
551   ltd330m040aaaaaaaaon   ltd330m040aaaaaaaaou
552   ltd330m080aaaaaaaaop   ltd330m080aaaaaaaaou
553   ltd330m080aaaaaaaaon   ltd330m080aaaaaaaaou
554   ltd330m120aaaaaaaaop   ltd330m120aaaaaaaaou
555   ltd330m120aaaaaaaaon   ltd330m120aaaaaaaaou
556   ltd330mr50aaaaaaaaop   ltd330mr50aaaaaaaaou
557   ltd330mr50aaaaaaaaon   ltd330mr50aaaaaaaaou
558   ltd330s020aaaaaaaaop   ltd330s020aaaaaaaaou
559   ltd330s020aaaaaaaaon   ltd330s020aaaaaaaaou
560   ltd330s040aaaaaaaaop   ltd330s040aaaaaaaaou
561   ltd330s040aaaaaaaaon   ltd330s040aaaaaaaaou
562   ltd330s080aaaaaaaaop   ltd330s080aaaaaaaaou
563   ltd330s080aaaaaaaaon   ltd330s080aaaaaaaaou
564   ltd330s120aaaaaaaaop   ltd330s120aaaaaaaaou
565   ltd330s120aaaaaaaaon   ltd330s120aaaaaaaaou
566   ltd330sr50aaaaaaaaop   ltd330sr50aaaaaaaaou
567   ltd330sr50aaaaaaaaon   ltd330sr50aaaaaaaaou
568   lvt330f020aaaaaaaaou   lvt330f020aaaaaaaaou
569   lvt330f040aaaaaaaaou   lvt330f040aaaaaaaaou
570   lvt330f080aaaaaaaaou   lvt330f080aaaaaaaaou
571   lvt330f120aaaaaaaaou   lvt330f120aaaaaaaaou
572   lvt330f160aaaaaaaaou   lvt330f160aaaaaaaaou
573   lvt330fr50aaaaaaaaou   lvt330fr50aaaaaaaaou
574   lvt330m020aaaaaaaaou   lvt330m020aaaaaaaaou
575   lvt330m040aaaaaaaaou   lvt330m040aaaaaaaaou
576   lvt330m080aaaaaaaaou   lvt330m080aaaaaaaaou
577   lvt330m120aaaaaaaaou   lvt330m120aaaaaaaaou
578   lvt330m160aaaaaaaaou   lvt330m160aaaaaaaaou
579   lvt330mr50aaaaaaaaou   lvt330mr50aaaaaaaaou
580   lvt330s020aaaaaaaaou   lvt330s020aaaaaaaaou
581   lvt330s040aaaaaaaaou   lvt330s040aaaaaaaaou
582   lvt330s080aaaaaaaaou   lvt330s080aaaaaaaaou
583   lvt330s120aaaaaaaaou   lvt330s120aaaaaaaaou
584   lvt330s160aaaaaaaaou   lvt330s160aaaaaaaaou
585   lvt330sr50aaaaaaaaou   lvt330sr50aaaaaaaaou
586   lvd330f020aaaaaaaaop   lvd330f020aaaaaaaaou
587   lvd330f020aaaaaaaaon   lvd330f020aaaaaaaaou
588   lvd330f040aaaaaaaaop   lvd330f040aaaaaaaaou
589   lvd330f040aaaaaaaaon   lvd330f040aaaaaaaaou
590   lvd330f080aaaaaaaaop   lvd330f080aaaaaaaaou
591   lvd330f080aaaaaaaaon   lvd330f080aaaaaaaaou
592   lvd330f120aaaaaaaaop   lvd330f120aaaaaaaaou
593   lvd330f120aaaaaaaaon   lvd330f120aaaaaaaaou
594   lvd330fr50aaaaaaaaop   lvd330fr50aaaaaaaaou
595   lvd330fr50aaaaaaaaon   lvd330fr50aaaaaaaaou
596   lvd330m020aaaaaaaaop   lvd330m020aaaaaaaaou
597   lvd330m020aaaaaaaaon   lvd330m020aaaaaaaaou
598   lvd330m040aaaaaaaaop   lvd330m040aaaaaaaaou
599   lvd330m040aaaaaaaaon   lvd330m040aaaaaaaaou
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[Diff pin]  inv_pin  vdiff  tdelay_typ  tdelay_min  tdelay_max
500   501   0.1   0.0s   0.0s   0.0s
502   503   0.1   0.0s   0.0s   0.0s
504   505   0.1   0.0s   0.0s   0.0s
506   507   0.1   0.0s   0.0s   0.0s
508   509   0.1   0.0s   0.0s   0.0s
510   511   0.1   0.0s   0.0s   0.0s
512   513   0.1   0.0s   0.0s   0.0s
514   515   0.1   0.0s   0.0s   0.0s
516   517   0.1   0.0s   0.0s   0.0s
518   519   0.1   0.0s   0.0s   0.0s
520   521   0.1   0.0s   0.0s   0.0s
522   523   0.1   0.0s   0.0s   0.0s
524   525   0.1   0.0s   0.0s   0.0s
526   527   0.1   0.0s   0.0s   0.0s
528   529   0.1   0.0s   0.0s   0.0s
530   531   0.1   0.0s   0.0s   0.0s
532   533   0.1   0.0s   0.0s   0.0s
534   535   0.1   0.0s   0.0s   0.0s
536   537   0.1   0.0s   0.0s   0.0s
538   539   0.1   0.0s   0.0s   0.0s
540   541   0.1   0.0s   0.0s   0.0s
542   543   0.1   0.0s   0.0s   0.0s
544   545   0.1   0.0s   0.0s   0.0s
546   547   0.1   0.0s   0.0s   0.0s
548   549   0.1   0.0s   0.0s   0.0s
550   551   0.1   0.0s   0.0s   0.0s
552   553   0.1   0.0s   0.0s   0.0s
554   555   0.1   0.0s   0.0s   0.0s
556   557   0.1   0.0s   0.0s   0.0s
558   559   0.1   0.0s   0.0s   0.0s
560   561   0.1   0.0s   0.0s   0.0s
562   563   0.1   0.0s   0.0s   0.0s
564   565   0.1   0.0s   0.0s   0.0s
566   567   0.1   0.0s   0.0s   0.0s
586   587   0.1   0.0s   0.0s   0.0s
588   589   0.1   0.0s   0.0s   0.0s
590   591   0.1   0.0s   0.0s   0.0s
592   593   0.1   0.0s   0.0s   0.0s
594   595   0.1   0.0s   0.0s   0.0s
596   597   0.1   0.0s   0.0s   0.0s
598   599   0.1   0.0s   0.0s   0.0s
600   601   0.1   0.0s   0.0s   0.0s
602   603   0.1   0.0s   0.0s   0.0s
604   605   0.1   0.0s   0.0s   0.0s
606   607   0.1   0.0s   0.0s   0.0s
608   609   0.1   0.0s   0.0s   0.0s
610   611   0.1   0.0s   0.0s   0.0s
612   613   0.1   0.0s   0.0s   0.0s
614   615   0.1   0.0s   0.0s   0.0s
866   867   NA   NA   NA   NA
868   869   NA   NA   NA   NA
870   871   NA   NA   NA   NA
872   873   NA   NA   NA   NA
874   875   NA   NA   NA   NA
876   877   NA   NA   NA   NA
878   879   NA   NA   NA   NA
880   881   NA   NA   NA   NA
882   883   NA   NA   NA   NA
884   885   NA   NA   NA   NA
886   887   NA   NA   NA   NA
888   889   NA   NA   NA   NA
890   891   NA   NA   NA   NA
892   893   NA   NA   NA   NA
894   895   NA   NA   NA   NA
896   897   NA   NA   NA   NA
898   899   NA   NA   NA   NA
900   901   NA   NA   NA   NA
902   903   NA   NA   NA   NA
904   905   NA   NA   NA   NA
906   907   NA   NA   NA   NA
908   909   NA   NA   NA   NA
910   911   NA   NA   NA   NA
912   913   NA   NA   NA   NA
914   915   NA   NA   NA   NA
916   917   NA   NA   NA   NA
918   919   NA   NA   NA   NA
920   921   NA   NA   NA   NA
922   923   NA   NA   NA   NA
924   925   NA   NA   NA   NA
926   927   NA   NA   NA   NA
928   929   NA   NA   NA   NA
930   931   NA   NA   NA   NA
932   933   NA   NA   NA   NA
934   935   NA   NA   NA   NA
936   937   NA   NA   NA   NA
938   939   NA   NA   NA   NA
940   941   NA   NA   NA   NA
942   943   NA   NA   NA   NA
944   945   NA   NA   NA   NA
946   947   NA   NA   NA   NA
948   949   NA   NA   NA   NA
950   951   NA   NA   NA   NA
952   953   NA   NA   NA   NA
954   955   NA   NA   NA   NA
956   957   NA   NA   NA   NA
958   959   NA   NA   NA   NA
960   961   NA   NA   NA   NA
962   963   NA   NA   NA   NA
964   965   NA   NA   NA   NA
966   967   NA   NA   NA   NA
968   969   NA   NA   NA   NA
970   971   NA   NA   NA   NA
972   973   NA   NA   NA   NA
974   975   NA   NA   NA   NA
976   977   NA   NA   NA   NA
978   979   NA   NA   NA   NA
980   981   NA   NA   NA   NA
982   983   NA   NA   NA   NA
984   985   NA   NA   NA   NA
986   987   0.1   0.0s   0.0s   0.0s
988   989   0.1   0.0s   0.0s   0.0s
1045   1046   0.1   0.0s   0.0s   0.0s
1047   1048   0.1   0.0s   0.0s   0.0s
1049   1050   0.1   0.0s   0.0s   0.0s
1051   1052   0.1   0.0s   0.0s   0.0s
1053   1054   0.1   0.0s   0.0s   0.0s
1055   1056   0.1   0.0s   0.0s   0.0s
1057   1058   0.1   0.0s   0.0s   0.0s
1059   1060   0.1   0.0s   0.0s   0.0s
1061   1062   0.1   0.0s   0.0s   0.0s
1063   1064   0.1   0.0s   0.0s   0.0s
1065   1066   0.1   0.0s   0.0s   0.0s
1067   1068   0.1   0.0s   0.0s   0.0s
1069   1070   0.1   0.0s   0.0s   0.0s
1071   1072   0.1   0.0s   0.0s   0.0s
1073   1074   0.1   0.0s   0.0s   0.0s
1075   1076   0.1   0.0s   0.0s   0.0s
1077   1078   0.1   0.0s   0.0s   0.0s
1079   1080   0.1   0.0s   0.0s   0.0s
1131   1132   0.1   0.0s   0.0s   0.0s
1133   1134   0.1   0.0s   0.0s   0.0s
1135   1136   0.1   0.0s   0.0s   0.0s
1137   1138   0.1   0.0s   0.0s   0.0s
1139   1140   0.1   0.0s   0.0s   0.0s
1141   1142   0.1   0.0s   0.0s   0.0s
1143   1144   0.1   0.0s   0.0s   0.0s
1145   1146   NA   NA   NA   NA
1147   1148   NA   NA   NA   NA
1149   1150   NA   NA   NA   NA
1151   1152   NA   NA   NA   NA
1153   1154   NA   NA   NA   NA
1155   1156   NA   NA   NA   NA
1157   1158   NA   NA   NA   NA
1159   1160   NA   NA   NA   NA
1221   1222   NA   NA   NA   NA
1223   1224   NA   NA   NA   NA
1273   1274   NA   NA   NA   NA
1275   1276   0.1   0.0s   0.0s   0.0s
1438   1439   NA   NA   NA   NA
1440   1441   NA   NA   NA   NA
1442   1443   NA   NA   NA   NA
1444   1445   NA   NA   NA   NA
1446   1447   NA   NA   NA   NA
1448   1449   NA   NA   NA   NA
1450   1451   NA   NA   NA   NA
1452   1453   NA   NA   NA   NA
1454   1455   NA   NA   NA   NA
1456   1457   NA   NA   NA   NA
1458   1459   NA   NA   NA   NA
1460   1461   NA   NA   NA   NA
1462   1463   NA   NA   NA   NA
1464   1465   NA   NA   NA   NA
1466   1467   NA   NA   NA   NA
1468   1469   NA   NA   NA   NA
1470   1471   NA   NA   NA   NA
1472   1473   NA   NA   NA   NA
1474   1475   NA   NA   NA   NA
1476   1477   NA   NA   NA   NA
1478   1479   NA   NA   NA   NA
1480   1481   NA   NA   NA   NA
1482   1483   NA   NA   NA   NA
1484   1485   NA   NA   NA   NA
1486   1487   NA   NA   NA   NA
1488   1489   NA   NA   NA   NA
1490   1491   NA   NA   NA   NA
1492   1493   NA   NA   NA   NA
1494   1495   NA   NA   NA   NA
1496   1497   NA   NA   NA   NA
1498   1499   NA   NA   NA   NA
1500   1501   NA   NA   NA   NA
1502   1503   NA   NA   NA   NA
1504   1505   NA   NA   NA   NA
1506   1507   NA   NA   NA   NA
1508   1509   NA   NA   NA   NA
1510   1511   NA   NA   NA   NA
1512   1513   NA   NA   NA   NA
1514   1515   NA   NA   NA   NA
1516   1517   NA   NA   NA   NA
1518   1519   NA   NA   NA   NA
1520   1521   NA   NA   NA   NA
1522   1523   NA   NA   NA   NA
1524   1525   NA   NA   NA   NA
1526   1527   NA   NA   NA   NA
1528   1529   NA   NA   NA   NA
1530   1531   NA   NA   NA   NA
1532   1533   NA   NA   NA   NA
1534   1535   NA   NA   NA   NA
1536   1537   NA   NA   NA   NA
1538   1539   NA   NA   NA   NA
1540   1541   NA   NA   NA   NA
1542   1543   NA   NA   NA   NA
1544   1545   NA   NA   NA   NA
1546   1547   NA   NA   NA   NA
1548   1549   NA   NA   NA   NA
1550   1551   NA   NA   NA   NA
1552   1553   NA   NA   NA   NA
1554   1555   NA   NA   NA   NA
1556   1557   NA   NA   NA   NA
1558   1559   NA   NA   NA   NA
1560   1561   NA   NA   NA   NA
1562   1563   NA   NA   NA   NA
1564   1565   NA   NA   NA   NA
1566   1567   NA   NA   NA   NA
1568   1569   NA   NA   NA   NA
1570   1571   NA   NA   NA   NA
1572   1573   NA   NA   NA   NA
1574   1575   NA   NA   NA   NA
1576   1577   NA   NA   NA   NA
1578   1579   NA   NA   NA   NA
1580   1581   NA   NA   NA   NA
1654   1655   NA   NA   NA   NA
1656   1657   NA   NA   NA   NA
1658   1659   NA   NA   NA   NA
1660   1661   NA   NA   NA   NA
1662   1663   NA   NA   NA   NA
1664   1665   NA   NA   NA   NA
1666   1667   NA   NA   NA   NA
1668   1669   NA   NA   NA   NA
1670   1671   NA   NA   NA   NA
1681   1682   0.1   0.0s   0.0s   0.0s
1683   1684   0.1   0.0s   0.0s   0.0s
1685   1686   0.1   0.0s   0.0s   0.0s
1687   1688   0.1   0.0s   0.0s   0.0s
1689   1690   0.1   0.0s   0.0s   0.0s
1691   1692   0.1   0.0s   0.0s   0.0s
1693   1694   0.1   0.0s   0.0s   0.0s
1695   1696   0.1   0.0s   0.0s   0.0s
1697   1698   0.1   0.0s   0.0s   0.0s
1699   1700   0.1   0.0s   0.0s   0.0s
1701   1702   0.1   0.0s   0.0s   0.0s
1703   1704   0.1   0.0s   0.0s   0.0s
1705   1706   0.1   0.0s   0.0s   0.0s
1707   1708   0.1   0.0s   0.0s   0.0s
[Series Pin Mapping]  pin_2   model_name   function_table_group
868   869   lvss
872   873   lvss
876   877   lvss
880   881   lvss
884   885   lvss
888   889   lvss
892   893   lvss
904   905   lvss
916   917   lvss
928   929   lvss
940   941   lvss
952   953   lvss
964   965   lvss
976   977   lvss
1133   1134   lvss
1135   1136   lvss
1139   1140   lvss
1143   1144   lvss
1147   1148   lvss
1151   1152   lvss
1155   1156   lvss
1159   1160   lvss
1221   1222   lvss
1223   1224   lvss
[Model]  lvss
Model_type   Series
C_comp   0  0  0
[Voltage Range]  1.8   1.75   1.85
[R Series]   100   110   90
|End [Model]
|End [Component]
| Models and submodels in the file (1480): lvt330f020eaaaaaaaio (I/O), lvt330f020faaaaaaaio (I/O), lvt330f020gaaaaaaaio (I/O), lvt330f020haaaaaaaio (I/O), lvt330f040eaaaaaaaio (I/O), lvt330f040faaaaaaaio (I/O), lvt330f040gaaaaaaaio (I/O), lvt330f040haaaaaaaio (I/O), lvt330f080eaaaaaaaio (I/O), lvt330f080faaaaaaaio (I/O), lvt330f080gaaaaaaaio (I/O), lvt330f080haaaaaaaio (I/O), lvt330f120eaaaaaaaio (I/O), lvt330f120faaaaaaaio (I/O), lvt330f120gaaaaaaaio (I/O), lvt330f120haaaaaaaio (I/O), lvt330f120iaaaaaaaio (I/O), lvt330f160eaaaaaaaio (I/O), lvt330f160faaaaaaaio (I/O), lvt330f160gaaaaaaaio (I/O), lvt330f160haaaaaaaio (I/O), lvt330fr50eaaaaaaaio (I/O), lvt330fr50faaaaaaaio (I/O), lvt330fr50gaaaaaaaio (I/O), lvt330fr50haaaaaaaio (I/O), lvt330m020eaaaaaaaio (I/O), lvt330m020faaaaaaaio (I/O), lvt330m020gaaaaaaaio (I/O), lvt330m020haaaaaaaio (I/O), lvt330m040eaaaaaaaio (I/O), lvt330m040faaaaaaaio (I/O), lvt330m040gaaaaaaaio (I/O), lvt330m040haaaaaaaio (I/O), lvt330m080eaaaaaaaio (I/O), lvt330m080faaaaaaaio (I/O), lvt330m080gaaaaaaaio (I/O), lvt330m080haaaaaaaio (I/O), lvt330m120eaaaaaaaio (I/O), lvt330m120faaaaaaaio (I/O), lvt330m120gaaaaaaaio (I/O), lvt330m120haaaaaaaio (I/O), lvt330m120iaaaaaaaio (I/O), lvt330m160eaaaaaaaio (I/O), lvt330m160faaaaaaaio (I/O), lvt330m160gaaaaaaaio (I/O), lvt330m160haaaaaaaio (I/O), lvt330mr50eaaaaaaaio (I/O), lvt330mr50faaaaaaaio (I/O), lvt330mr50gaaaaaaaio (I/O), lvt330mr50haaaaaaaio (I/O), lvt330s020eaaaaaaaio (I/O), lvt330s020faaaaaaaio (I/O), lvt330s020gaaaaaaaio (I/O), lvt330s020haaaaaaaio (I/O), lvt330s040eaaaaaaaio (I/O), lvt330s040faaaaaaaio (I/O), lvt330s040gaaaaaaaio (I/O), lvt330s040haaaaaaaio (I/O), lvt330s080eaaaaaaaio (I/O), lvt330s080faaaaaaaio (I/O), lvt330s080gaaaaaaaio (I/O), lvt330s080haaaaaaaio (I/O), lvt330s120eaaaaaaaio (I/O), lvt330s120faaaaaaaio (I/O), lvt330s120gaaaaaaaio (I/O), lvt330s120haaaaaaaio (I/O), lvt330s120iaaaaaaaio (I/O), lvt330s160eaaaaaaaio (I/O), lvt330s160faaaaaaaio (I/O), lvt330s160gaaaaaaaio (I/O), lvt330s160haaaaaaaio (I/O), lvt330sr50eaaaaaaaio (I/O), lvt330sr50faaaaaaaio (I/O), lvt330sr50gaaaaaaaio (I/O), lvt330sr50haaaaaaaio (I/O), lvt330f020aaaaaaaaod (I/O_open_drain), lvt330f040aaaaaaaaod (I/O_open_drain), lvt330f080aaaaaaaaod (I/O_open_drain), lvt330f120aaaaaaaaod (I/O_open_drain), lvt330m020aaaaaaaaod (I/O_open_drain)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
